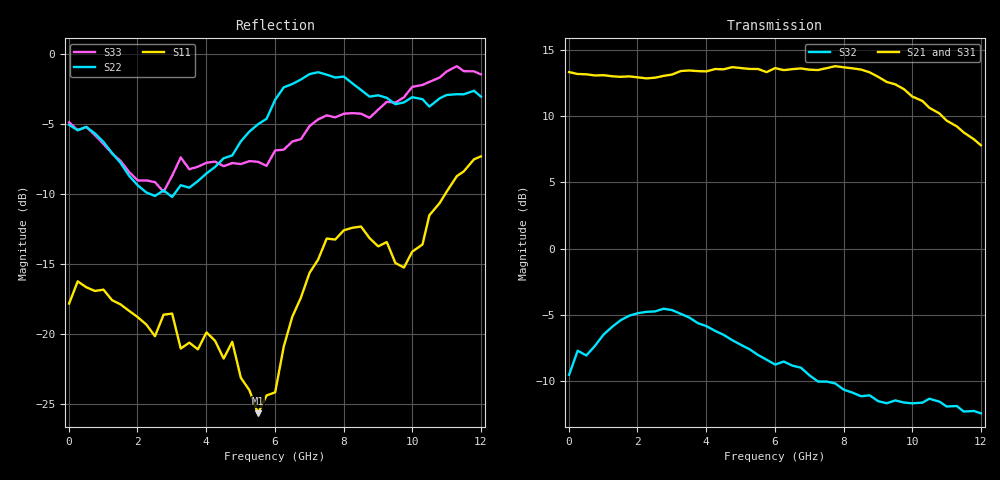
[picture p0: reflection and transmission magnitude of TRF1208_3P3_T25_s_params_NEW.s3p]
! Created Thu Mar  3 20:30:45 2022
# hz S ri R 50
! 3 Port Network Data from SP1.SP block
! freq  reS11  imS11  reS12  imS12  reS13  imS13
!  reS21  imS21
!  reS22  imS22  reS23  imS23
!  reS31  imS31  reS32  imS32
!  reS33  imS33
! Terminal data exported
! Port[1] = INP
! Port[2] = OUTP
! Port[3] = OUTM
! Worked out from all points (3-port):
!   49 points, 10 MHz to 12 GHz, reference 50 ohm
!   strongest paths, dB at 10 MHz, 3.01 GHz, 6.01 GHz, 9.01 GHz, 12 GHz:
!     S21: 13.3, 13.1, 13.6, 13.0, 7.8
!     S31: 13.1, 13.1, 13.7, 13.0, 7.8
!     S32: -9.5, -4.6, -8.8, -11.5, -12.4
!   lowest |S11| = -25.6 dB at 5.51 GHz (marker M1), VSWR 1.11, Z = 45.3 + j1.75 ohm
!   |S11| at or under -10 dB: start of sweep to 10.96 GHz
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1e7  -0.1254 -0.0285  0.0686 -0.00456  0.0523 0.00167
     -4.639 -0.0221  -0.5568 -0.0181  0.3603 0.0219
     4.524 0.00291  0.3343 0.00678  -0.5685 -0.0255
1.51e9  -0.1204 0.0425  0.0943 0.00752  0.0851 0.00111
        -3.959 2.036  -0.3559 0.1984  0.5507 -0.0222
        3.947 -2.03  0.5365 -0.0245  -0.3607 0.2034
3.26e9  -0.0864 0.021  0.1148 -0.0376  0.1001 -0.0523
        -2.825 3.735  -0.3394 0.00552  0.5343 -0.4019
        2.773 -3.778  0.4692 -0.3195  -0.4154 0.097
4.76e9  -0.0914 -0.0218  0.1006 -0.088  0.074 -0.104
        -0.9532 4.748  -0.4316 0.0402  0.1483 -0.5782
        0.9121 -4.705  0.2586 -0.3701  -0.3425 0.2205
5.51e9  -0.0486 0.0193  0.0726 -0.1079  0.0366 -0.1247
        0.3892 4.752  -0.4978 0.2558  -0.1164 -0.4875
        -0.3539 -4.74  0.1521 -0.3667  -0.2369 0.3364
6.01e9  -0.0411 0.0466  0.0538 -0.1157  0.009 -0.1249
        1.052 4.686  -0.5718 0.3763  -0.2252 -0.3772
        -1.076 -4.697  0.1118 -0.3476  -0.2182 0.3953
7.76e9  0.0882 0.1988  0.00699 -0.0955  -0.0548 -0.0841
        3.576 3.328  -0.4296 0.7  -0.2047 -0.0264
        -3.54 -3.136  -0.1466 -0.273  -0.324 0.4962
8.76e9  0.1094 0.1907  -0.00193 -0.0891  -0.0663 -0.0585
        4.347 1.595  -0.1671 0.682  -0.1513 0.0398
        -4.329 -1.593  -0.2584 -0.1066  -0.2502 0.5347
1.03e10  -0.097 0.185  -0.0241 -0.0786  -0.0645 -0.0209
         3.47 -0.9899  0.0974 0.6806  -0.1009 0.1125
         -3.47 1.011  -0.1721 0.1981  0.0242 0.7726
1.2e10  -0.3751 0.2103  -0.0361 -0.0537  -0.054 0.00505
        1.783 -1.69  -0.2005 0.6731  -0.0692 0.1674
        -1.857 1.612  -0.00232 0.2391  -0.1932 0.8207
